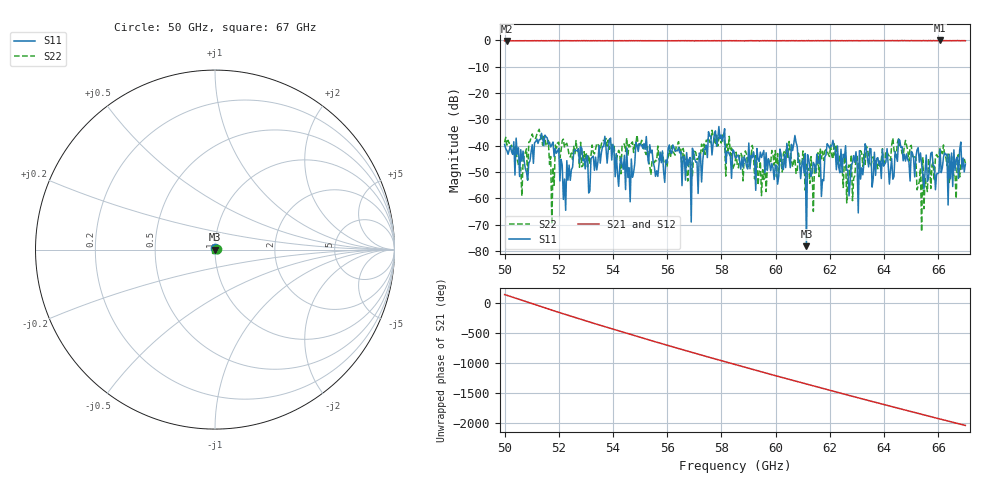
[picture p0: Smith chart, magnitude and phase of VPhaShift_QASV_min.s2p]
!Agilent Technologies,E8361A,US42410132,A.06.03.05
!Agilent E8361A: A.06.03.05
!Date: Friday, July 11, 2008 15:24:53
!Correction: S11(Full 2 Port(1,2)) S21(Full 2 Port(1,2)) S12(Full 2 Port(1,2)) S22(Full 2 Port(1,2))
!S2P File: Measurements: S11, S21, S12, S22:
# Hz S  MA  R 50
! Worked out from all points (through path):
!   401 points, 50 GHz to 67 GHz, reference 50 ohm
!   highest |S21| = -0.11 dB at 66.06 GHz (marker M1); lowest = -0.3 dB at 50.09 GHz (marker M2)
!   lowest |S11| = -78.2 dB at 61.13 GHz (marker M3), VSWR 1.00, Z = 50 + j0.0106 ohm
!   |S11| at or under -10 dB: start of sweep to end of sweep
!   |S22| runs from -72.7 to -33.8 dB; largest |S21 - S12| = 0.018
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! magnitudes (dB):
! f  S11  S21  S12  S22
! 50 GHz  -39.6  -0.3  -0.2  -38.8
! 50.09 GHz  -41.9  -0.3  -0.2  -39.9
! 50.59 GHz  -41.6  -0.2  -0.2  -48.3
! 51.27 GHz  -37.8  -0.2  -0.2  -33.8
! 51.74 GHz  -39.7  -0.3  -0.2  -69.9
! 52.25 GHz  -64.6  -0.2  -0.1  -39.6
! 52.85 GHz  -41.0  -0.2  -0.2  -48.0
! 55.7 GHz  -47.3  -0.3  -0.2  -45.4
! 56.84 GHz  -44.5  -0.2  -0.2  -45.4
! 57.73 GHz  -36.1  -0.2  -0.3  -37.6
! 58.5 GHz  -44.4  -0.2  -0.2  -46.7
! 60.03 GHz  -47.6  -0.2  -0.2  -51.8
! 60.67 GHz  -39.4  -0.2  -0.2  -46.1
! 61.13 GHz  -78.2  -0.2  -0.2  -47.1
! 61.35 GHz  -49.8  -0.2  -0.2  -50.3
! 62.03 GHz  -40.1  -0.2  -0.2  -39.8
! 62.71 GHz  -59.1  -0.2  -0.2  -47.3
! 64.19 GHz  -54.6  -0.2  -0.2  -44.1
! 65.05 GHz  -42.9  -0.2  -0.2  -44.3
! 65.47 GHz  -56.4  -0.2  -0.2  -64.0
! 66.06 GHz  -41.4  -0.1  -0.2  -41.1
! 67 GHz  -47.0  -0.2  -0.3  -46.7
